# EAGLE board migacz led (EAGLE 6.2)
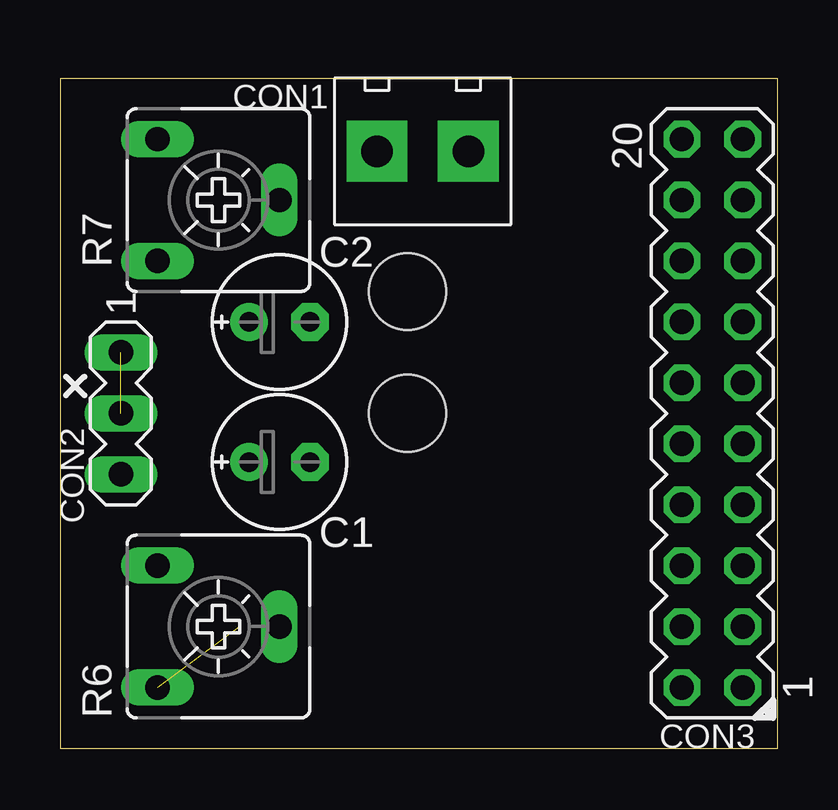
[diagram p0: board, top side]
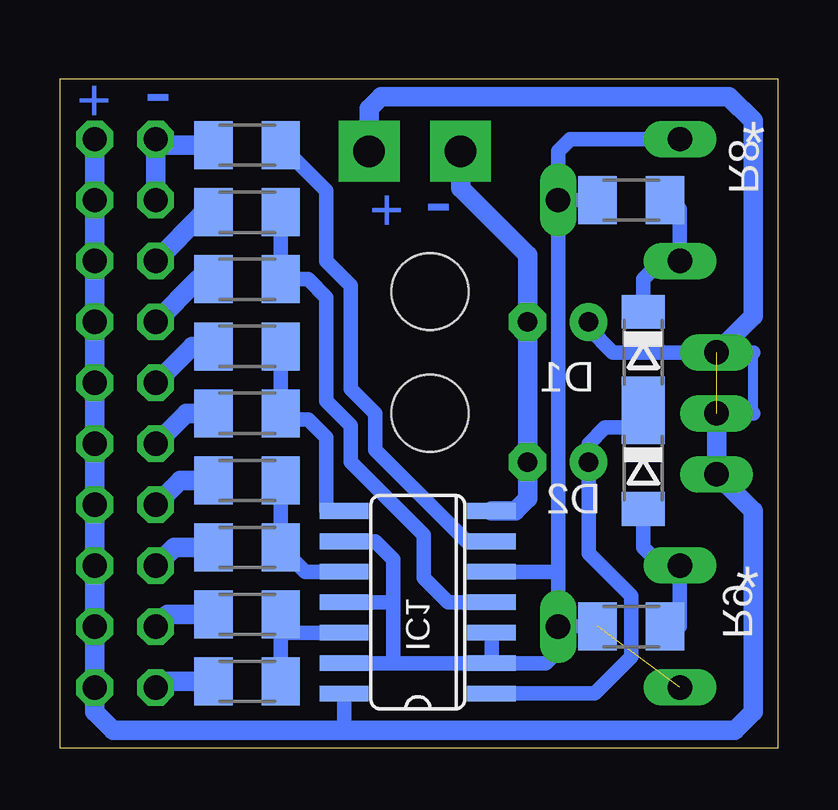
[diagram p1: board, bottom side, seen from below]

Size 29.9 x 27.93 mm. Coordinates in mm from the lower left corner, seen from the top.
Outline: 0,0 29.9,0 29.9,27.93 0,27.93 0,0
Copper layers (1*16): Top 0.035mm / dielectric 1.5mm / Bottom 0.035mm
Design rules: minimum track width 10mil, minimum drill 24mil, track to track 8mil, track to pad 8mil, pad to pad 8mil, via to via 8mil, smd to smd 8mil, copper to edge 40mil, drill to drill 8mil, minimum pad ring 10mil, minimum via ring 8mil, stop-mask expansion 4mil, vias tented up to drill 0mil, thermal gap 10mil
Holes 3.2 mm at 14.48,13.97 14.48,19.05

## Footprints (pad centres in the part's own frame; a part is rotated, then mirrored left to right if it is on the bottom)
E2,5-6E = drill 0.813 pad 1.575: + -1.27,0 | drill 0.813 pad 1.575 octagon: - 1.27,0
ARK300/2 = drill 1.3 pad 2.54 square: 1 -1.27,0; 2 2.54,0
MA03-1 = drill 1.016 long: 1 -2.54,0; 2 0,0; 3 2.54,0
MA10-2 = drill 1.016 octagon: 1 -11.43,-1.27; 2 -11.43,1.27; 3 -8.89,-1.27; 4 -8.89,1.27; 5 -6.35,-1.27; 6 -6.35,1.27; 7 -3.81,-1.27; 8 -3.81,1.27; 9 -1.27,-1.27; 10 -1.27,1.27; 11 1.27,-1.27; 12 1.27,1.27; 13 3.81,-1.27; 14 3.81,1.27; 15 6.35,-1.27; 16 6.35,1.27; 17 8.89,-1.27; 18 8.89,1.27; 19 11.43,-1.27; 20 11.43,1.27
SOD80C = smd 1.4 x 1.8: A 1.7,0; C -1.7,0
SO14 = smd 0.66 x 2.032: 1 -3.81,-3.073; 2 -2.54,-3.073; 3 -1.27,-3.073; 4 0,-3.073; 5 1.27,-3.073; 6 2.54,-3.073; 7 3.81,-3.073; 8 3.81,3.073; 9 2.54,3.073; 10 1.27,3.073; 11 0,3.073; 12 -1.27,3.073; 13 -2.54,3.073; 14 -3.81,3.073
M1206 = smd 1.6 x 2: 1 -1.4,0; 2 1.4,0
CA6V = drill 1.016 long: A -2.54,-2.54; E 2.54,-2.54; S 0,2.54

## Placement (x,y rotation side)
C1  22uF  [E2,5-6E]  9.14,11.94 0 top
C2  22uF  [E2,5-6E]  9.14,17.78 0 top
CON1  [ARK300/2]  14.48,24.89 0 top
CON2  [MA03-1]  2.54,13.97 270 top
CON3  [MA10-2]  27.18,13.97 90 top
D1  4148  [SOD80C]  5.59,16.51 270 bottom
D2  4148  [SOD80C]  5.59,11.68 270 bottom
IC1  40106D  [SO14]  14.99,6.1 90 bottom
R1  [M1206]  22.1,25.15 180 bottom
R2  [M1206]  22.1,22.35 180 bottom
R3  [M1206]  22.1,19.56 180 bottom
R4  [M1206]  22.1,16.76 180 bottom
R5  [M1206]  22.1,13.97 180 bottom
R6  500k  [CA6V]  6.6,5.08 270 top
R7  500k  [CA6V]  6.6,22.86 270 top
R8  *  [M1206]  6.1,22.86 180 bottom
R9  *  [M1206]  6.1,5.08 180 bottom
R10  [M1206]  22.1,11.18 180 bottom
R11  [M1206]  22.1,8.38 180 bottom
R12  [M1206]  22.1,5.59 180 bottom
R13  [M1206]  22.1,2.79 180 bottom

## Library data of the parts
C1 C2 R1-R5 R8-R13 = rcl
CON1 = DS
CON2 CON3 = con-lstb
D1 D2 = diode
IC1 = 40xx
R6 R7 = pot

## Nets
GND: C1.- C2.- CON1.1 IC1.7
N$1: C2.+ CON2.2 CON2.3 CON3.1 CON3.3 CON3.5 CON3.7 CON3.9 CON3.11 CON3.13 CON3.15 CON3.17 CON3.19 IC1.14
N$2: CON3.18 CON3.20 R1.2
N$3: CON3.16 R2.2
N$4: CON3.12 R4.2
N$5: CON3.6 R11.2
N$6: CON3.2 R13.2
N$7: IC1.6 R1.1
N$8: IC1.4 R2.1 R3.1
N$9: IC1.8 R4.1 R5.1
N$10: IC1.10 R10.1 R11.1
N$11: IC1.12 R12.1 R13.1
N$12: CON1.2 CON2.1
N$13: CON3.4 R12.2
N$14: C1.+ D1.A D2.C IC1.1
N$15: D1.C R7.E R8.1
N$16: D2.A R6.A R9.1
N$17: IC1.2 IC1.3 IC1.5 IC1.9 IC1.11 IC1.13 R6.E R6.S R7.A R7.S R8.2 R9.2
N$18: CON3.8 R10.2
N$19: CON3.10 R5.2
N$20: CON3.14 R3.2

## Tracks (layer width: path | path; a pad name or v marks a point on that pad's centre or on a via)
GND
  Bottom 0.813: CON1.1 13.21,23.37 10.41,20.57 C2.- C1.- 10.41,10.41 10.92,9.91 IC1.7
N$1  (1 unrouted)
  Bottom 0.61: IC1.14 18.06,1.04 17.78,0.76 | C2.+ 7.87,17.53 6.86,16.51 2.54,16.51
  Bottom 0.813: CON3.19 CON3.17 CON3.15 CON3.13 CON3.11 CON3.9 CON3.7 CON3.5 CON3.3 CON3.1 28.45,1.52 27.69,0.76 17.78,0.76 1.78,0.76 1.02,1.52 1.02,9.91 CON2.3 CON2.2
N$2
  Bottom 0.813: CON3.18 CON3.20 25.65,25.15 R1.2
N$3
  Bottom 0.813: R2.2 23.88,22.35 CON3.16
N$4
  Bottom 0.813: R4.2 24.38,16.76 CON3.12
N$5
  Bottom 0.813: R11.2 25.15,8.38 CON3.6
N$6
  Bottom 0.813: R13.2 25.65,2.79 CON3.2
N$7
  Bottom 0.61: IC1.6 12.95,8.64 16.76,12.45 16.76,13.97 17.78,14.99 17.78,19.3 18.8,20.32 18.8,23.24 R1.1
N$8
  Bottom 0.61: IC1.4 13.72,6.1 14.73,7.11 14.73,8.89 17.78,11.94 17.78,13.46 18.8,14.48 18.8,18.8 19.56,19.56 R3.1 R2.1
N$9
  Bottom 0.61: R4.1 R5.1 20.44,13.72 19.56,13.72 18.8,12.95 18.8,9.91 IC1.8
N$10
  Bottom 0.61: R10.1 R11.1 19.68,7.37 IC1.10
N$11
  Bottom 0.61: 20.7,4.83 R13.1 | 20.7,4.83 R12.1 | IC1.12 20.7,4.83
N$12
  Bottom 0.406: 1.02,13.97 1.02,16.51
  Bottom 0.61: 1.02,16.51 CON2.1 | 1.02,13.97 2.29,13.97
  Bottom 0.813: CON1.2 17.02,26.67 16.51,27.18 2.03,27.18 1.02,26.16 1.02,18.03 CON2.1
N$13
  Bottom 0.813: R12.2 25.4,5.59 CON3.4
N$14
  Bottom 0.61: IC1.1 7.62,2.29 6.1,3.81 6.1,6.35 7.87,8.13 C1.+ 7.87,12.7 7.19,13.38 D2.C D1.A
N$15
  Bottom 0.61: R8.1 4.06,22.48 R7.E 4.83,20.32 5.59,19.56 D1.C
N$16
  Bottom 0.61: R9.1 4.06,5.08 R6.A 4.83,7.62 5.59,8.38 D2.A
N$17  (1 unrouted)
  Bottom 0.61: IC1.9 16.76,8.64 16,7.87 16,6.1 | 16,3.56 16,6.1 | 16,3.56 IC1.13 | 16,6.1 IC1.11 | IC1.2 16,3.56 | IC1.2 IC1.3 | IC1.2 9.65,3.56 9.14,4.06 R6.S | R6.S R9.2 | R7.A 8.64,25.4 9.14,24.89 R7.S | R7.S R8.2 | R6.S 9.14,7.37 | 9.14,7.37 R7.S | 9.14,7.37 IC1.5
N$18
  Bottom 0.813: R10.2 24.89,11.18 CON3.8
N$19
  Bottom 0.813: R5.2 24.64,13.97 CON3.10
N$20
  Bottom 0.813: R3.2 24.13,19.56 CON3.14

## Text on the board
Bottom: - | + | - | +
tPlace: CON1 | CON2 | CON3
bNames: * | * | IC1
